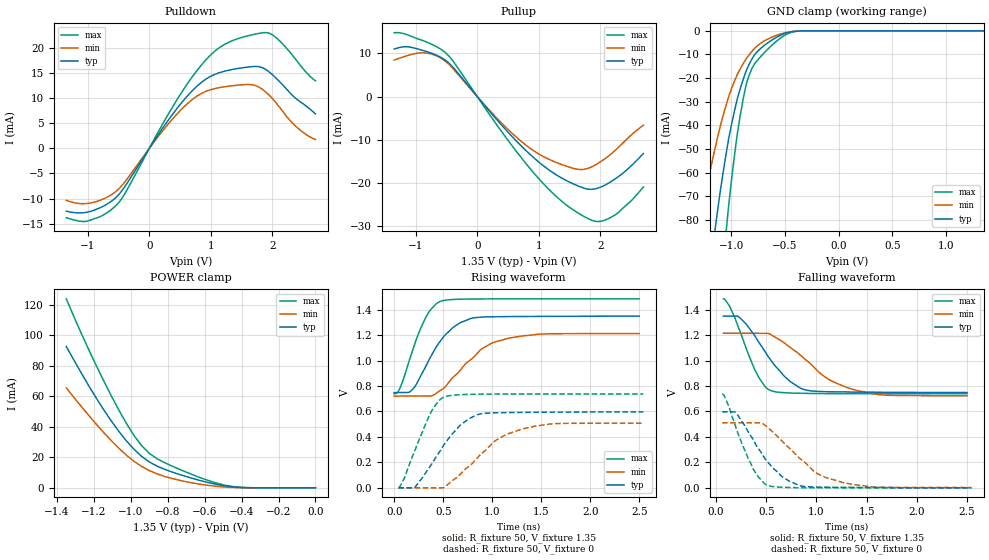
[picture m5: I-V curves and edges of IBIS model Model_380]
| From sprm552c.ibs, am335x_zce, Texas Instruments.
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| Model based on original model for BCSHTLTCSCDVPBFZ_SSDHV
|   Sub model SR11_6MA_10PER_1P35
[model]   Model_380
|[Description]  [1.35V-3-STATE-NOTERM-SR11:6MA, IND, 10%]
|   Slowest slew rate (SR[1:0] = "11"), 1.33 * RExt = 0.750 * Iout
|   (I[2:0] = "001"), 6mA nominal with Rext = 50R,ODT off (ODT[1:0]
|   = "00") CMOS mode,Industrial temperature range (-40C to 125C,
|   25C nominal),10% power supply tolerance
|[Input Load]   NOTERM
|[Output Drive] SR11:6MA
|Voltage   1.35V
|Mode   3-STATE
Model_type   3-state
Polarity   Non-Inverting
Enable   Active-Low
Cref =  15pF
Rref =  100.0000M
Vref =  0V
Vmeas =  0.675
C_comp   1.865048p   1.676829p   1.989968p
[Temperature Range]   25   125   -40
[Voltage Range]   1.35   1.215   1.485
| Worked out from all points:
|   slope of the pulldown table from 0 to 0.203 V, typ, clamps not added: 53.9 ohm
|   slope of the pullup table from 0 to 0.203 V, typ, clamps not added: 58.7 ohm
|   GND clamp passes 1 mA (typ) near -0.49 V on its own axis
|   POWER clamp passes 1 mA (typ) near -0.47 V on its own axis
|   rising waveform, R_fixture 50, V_fixture 1.35: 20-80 % time 297ps typ, 396ps min, 211ps max; typ from 0.749 V to 1.35 V
|   rising waveform, R_fixture 50, V_fixture 0: 20-80 % time 334ps typ, 445ps min, 236ps max; typ from 0 V to 0.597 V
|   falling waveform, R_fixture 50, V_fixture 1.35: 20-80 % time 337ps typ, 486ps min, 223ps max; typ from 1.35 V to 0.748 V
|   falling waveform, R_fixture 50, V_fixture 0: 20-80 % time 325ps typ, 423ps min, 223ps max; typ from 0.597 V to 0 V
[POWER_clamp]
-1.35V    92.75mA    65.6mA     124mA
-1.227V   66.81mA    47.39mA    90.41mA
-1.145V   50.92mA    36.05mA    69.79mA
-1.064V   36.83mA    25.81mA    50.69mA
-981.8mV  25.17mA    17.34mA    34.13mA
-940.9mV  20.58mA    14.01mA    27.55mA
-900mV    17mA       11.33mA    22.63mA
-859.1mV  14.3mA     9.219mA    19.19mA
-736.4mV  8.769mA    4.944mA    12.14mA
-490.9mV  1.299mA    528.4uA    1.73mA
-368.2mV  117.2uA    50.88uA    117.5uA
0V        1.028nA    11.64nA    1.384nA
[Pulldown]
-1.35V    -12.46mA   -10.34mA   -13.78mA
-1.023V   -12.73mA   -10.98mA   -14.51mA
-531.8mV  -9.642mA   -8.454mA   -11.24mA
-409.1mV  -7.802mA   -6.854mA   -9.239mA
204.5mV   3.794mA    3.288mA    4.579mA
572.7mV   9.763mA    8.353mA    12mA
900mV     13.58mA    11.21mA    17.32mA
1.227V    15.34mA    12.24mA    20.68mA
1.677V    16.25mA    12.62mA    22.57mA
1.964V    15.02mA    10.36mA    22.79mA
2.373V    9.983mA    4.461mA    17.78mA
2.7V      6.853mA    1.749mA    13.41mA
[Pullup]
-1.35V    11.03mA    8.458mA    14.78mA
-1.145V   11.56mA    9.461mA    14.36mA
-859.1mV  10.61mA    10.14mA    12.86mA
-490.9mV  8.13mA     7.885mA    9.838mA
286.4mV   -4.838mA   -4.502mA   -5.924mA
736.4mV   -11.73mA   -10.62mA   -14.53mA
1.227V    -17.6mA    -14.93mA   -22.38mA
1.636V    -20.69mA   -16.86mA   -26.96mA
1.923V    -21.35mA   -15.82mA   -28.91mA
2.086V    -20.44mA   -14.29mA   -28.55mA
2.291V    -18.58mA   -11.81mA   -26.9mA
2.7V      -13.18mA   -6.641mA   -20.95mA
[GND_clamp]
-1.35V    -159.1mA   -94.77mA   -266.2mA
-1.295V   -137.7mA   -81.77mA   -230.9mA
-1.159V   -87.19mA   -51.56mA   -145.9mA
-1.132V   -77.89mA   -46.14mA   -129.9mA
-1.05V    -52.83mA   -31.83mA   -86.44mA
-1.023V   -45.55mA   -27.75mA   -73.68mA
-940.9mV  -28.44mA   -18.28mA   -42.92mA
-859.1mV  -16.79mA   -11.75mA   -22.47mA
-804.5mV  -11.72mA   -8.559mA   -15.69mA
-722.7mV  -7.324mA   -5.161mA   -10.76mA
-395.5mV  -159.1uA   -161.1uA   -232.4uA
1.35V     1.028nA    146.6nA    745.7pA
[Ramp]
dV/dt_f 0.36256263/0.33920452n 0.29854988/0.49557384n  0.4483239/0.22412824n
dV/dt_r 0.36034268/0.33572213n 0.30915697/0.45294433n 0.44375724/0.23606605n
R_load = 50
[Rising Waveform]
R_fixture = 50
V_fixture = 1.35
V_fixture_min = 1.215
V_fixture_max = 1.485
0s        748.5mV    720.6mV    740.2mV
60.22ps   748.9mV    720.6mV    786.4mV
196.9ps   782.1mV    721mV      1.101V
330.7ps   968.7mV    721.6mV    1.352V
470.9ps   1.154V     765.7mV    1.465V
681.8ps   1.3V       931.8mV    1.483V
881.6ps   1.341V     1.085V     1.485V
1.026ns   1.345V     1.146V     1.485V
1.482ns   1.347V     1.208V     1.485V
2.5ns     1.349V     1.213V     1.485V
[Rising Waveform]
R_fixture = 50
V_fixture = 0
V_fixture_min = 0
V_fixture_max = 0
42.57ps   0V         0V         0V
204.7ps   0V         0V         280.9mV
370.2ps   171.8mV    0V         587.3mV
510.8ps   342.7mV    4.654mV    714.2mV
673.3ps   491.8mV    106mV      731.9mV
833.6ps   570.9mV    222.8mV    735.6mV
1.035ns   590mV      372.2mV    737mV
1.29ns    593mV      459.3mV    737.5mV
1.639ns   595mV      504.3mV    737.7mV
2.543ns   597.1mV    508.5mV    737.7mV
[Falling Waveform]
R_fixture = 50
V_fixture = 1.35
V_fixture_min = 1.215
V_fixture_max = 1.485
73.95ps   1.349V     1.214V     1.484V
139ps     1.349V     1.214V     1.421V
236.4ps   1.336V     1.214V     1.237V
414.4ps   1.158V     1.214V     883.6mV
545.9ps   1.004V     1.204V     764mV
858.7ps   776.6mV    1.028V     742.2mV
1.1ns     755.3mV    862.8mV    740mV
1.327ns   752.6mV    782.1mV    739.4mV
1.672ns   750.5mV    728.6mV    739.2mV
2.5ns     748.5mV    723mV      739.2mV
[Falling Waveform]
R_fixture = 50
V_fixture = 0
V_fixture_min = 0
V_fixture_max = 0
60.93ps   597.3mV    511.1mV    736.8mV
125.2ps   597.3mV    511.1mV    646mV
203.1ps   585.6mV    511.1mV    460.8mV
371.9ps   376.4mV    511.1mV    145.8mV
513.5ps   204.7mV    475.2mV    19.81mV
820.3ps   20.52mV    241.3mV    0V
1.003ns   6.174mV    115.1mV    0V
1.234ns   4.12mV     47.49mV    0V
1.595ns   2.645mV    5.649mV    0V
2.543ns   0V         2.577mV    0V
